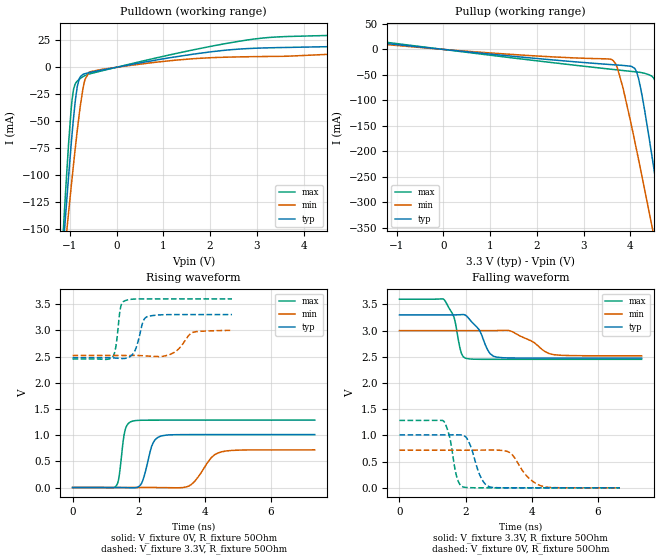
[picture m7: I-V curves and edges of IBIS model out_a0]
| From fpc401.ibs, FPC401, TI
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|   out_a0 Model
[Model]   out_a0
Model_type   Output
Polarity   Non-Inverting
Vmeas = 1.65
Vref = 0
Cref = 2pF
Rref = 5000
|   typ   min   max
|   (nom PVT)   (fast PVT)   (slow PVT)
C_comp   1.198e-12   1.173e-12   1.252e-12
| Where nom  PVT is Nominal Process, 3.3V, 27C
|   Fast PVT is Strong Process,  3.6V, -40C
|   Slow PVT is Weak Process,   3V, 125C
[Voltage Range]   3.3   3   3.6
|Junction Temperature
[Temperature Range]   27   125   -40
[Pullup Reference]   3.3   3   3.6
[Pulldown Reference]   0   0   0
[Power Clamp Reference]   3.3   3   3.6
[GND Clamp Reference]   0   0   0
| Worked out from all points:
|   slope of the pulldown table from 0 to 0.495 V, typ, clamps not added: 123 ohm
|   slope of the pullup table from 0 to 0.495 V, typ, clamps not added: 108 ohm
|   falling waveform, V_fixture 3.3V, R_fixture 50Ohm: 20-80 % time 426ps typ, 735ps min, 267ps max; typ from 3.3 V to 2.48 V
|   rising waveform, V_fixture 0V, R_fixture 50Ohm: 20-80 % time 249ps typ, 477ps min, 149ps max; typ from 0 V to 1.01 V
|   rising waveform, V_fixture 3.3V, R_fixture 50Ohm: 20-80 % time 209ps typ, 359ps min, 127ps max; typ from 2.48 V to 3.3 V
|   falling waveform, V_fixture 0V, R_fixture 50Ohm: 20-80 % time 317ps typ, 509ps min, 220ps max; typ from 1.01 V to 0 V
[Pulldown]
|   Voltage   I(typ)   I(min)   I(max)
-3.3V     -1.546A    -1.218A    -1.953A
-1.218V   -213.8mA   -220.6mA   -213.2mA
-1.115V   -152.3mA   -174.1mA   -133.9mA
-1.028V   -102.8mA   -136.1mA   -72.62mA
-924mV    -48.82mA   -91.83mA   -21.53mA
-838.2mV  -17.45mA   -58mA      -12.7mA
-696.3mV  -6.201mA   -15.06mA   -8.129mA
-582mV    -4.84mA    -4.296mA   -6.15mA
-330mV    -2.716mA   -2.011mA   -3.428mA
2.993V    17.77mA    9.963mA    26.56mA
4.584V    19.24mA    12.17mA    29.68mA
6.6V      33.13mA    35.22mA    33.6mA
[Pullup]
|   Voltage   I(typ)   I(min)   I(max)
-3.3V     32.44mA    31.14mA    37.81mA
3.585V    -29.8mA    -19.58mA   -38.89mA
3.726V    -30.71mA   -37.64mA   -40.28mA
4.029V    -33.53mA   -151.9mA   -43.21mA
4.175V    -56.83mA   -215.8mA   -44.69mA
4.454V    -204.9mA   -343.1mA   -52.13mA
4.518V    -242.7mA   -372.4mA   -59.95mA
4.591V    -287.3mA   -406.4mA   -92mA
4.663V    -331.4mA   -439.9mA   -139.5mA
4.749V    -384.4mA   -480mA     -203.1mA
4.937V    -501.6mA   -568mA     -351.5mA
6.6V      -1.559A    -1.368A    -1.735A
[Ramp]
R_load = 50
|   typ   min   max
dV/dt_r   0.605937/2.48756e-10   0.43132/4.77459e-10   0.77163/1.48535e-10
dV/dt_f   0.494035/4.25837e-10   0.288182/7.36969e-10   0.688486/2.66857e-10
[Falling Waveform]
V_fixture = 3.3V
V_fixture_min = 3V
V_fixture_max = 3.6V
R_fixture = 50Ohm
|   Time   V(typ)   V(min)   V(max)
0s        3.3V       3V         3.6V
1.352ns   3.3V       3V         3.591V
1.653ns   3.301V     3V         3.251V
1.877ns   3.305V     3V         2.561V
2.038ns   3.274V     3V         2.468V
2.433ns   2.993V     3V         2.453V
2.739ns   2.562V     3V         2.453V
2.951ns   2.494V     3.002V     2.453V
4.654ns   2.477V     2.542V     2.453V
7.325ns   2.477V     2.52V      2.453V
[Rising Waveform]
V_fixture = 0V
V_fixture_min = 0V
V_fixture_max = 0V
R_fixture = 50Ohm
|   Time   V(typ)   V(min)   V(max)
0s        1.218nV    15.44nV    982.1pV
1.311ns   439.2uV    480.9nV    25.22mV
1.586ns   -1.725mV   -17.86uV   1.089V
1.831ns   -5.716mV   27.74uV    1.27V
2.095ns   91.16mV    274.3uV    1.284V
2.39ns    782.6mV    301.2uV    1.286V
2.661ns   978.8mV    -772.7uV   1.286V
3.525ns   1.01V      30.92mV    1.286V
4.515ns   1.01V      682.6mV    1.286V
7.325ns   1.01V      718.9mV    1.286V
[Rising Waveform]
V_fixture = 3.3V
V_fixture_min = 3V
V_fixture_max = 3.6V
R_fixture = 50Ohm
|   Time   V(typ)   V(min)   V(max)
0s        2.477V     2.52V      2.453V
1.217ns   2.475V     2.52V      2.497V
1.311ns   2.47V      2.52V      2.695V
1.447ns   2.463V     2.52V      3.422V
1.586ns   2.464V     2.52V      3.565V
1.879ns   2.602V     2.52V      3.597V
2.257ns   3.26V      2.51V      3.6V
3.061ns   3.3V       2.573V     3.6V
3.634ns   3.3V       2.959V     3.6V
4.822ns   3.3V       2.999V     3.6V
[Falling Waveform]
V_fixture = 0V
V_fixture_min = 0V
V_fixture_max = 0V
R_fixture = 50Ohm
|   Time   V(typ)   V(min)   V(max)
0s        1.01V      718.9mV    1.286V
1.332ns   1.01V      718.9mV    1.277V
1.531ns   1.011V     718.9mV    934.8mV
1.753ns   1.012V     718.8mV    167.1mV
1.93ns    1.003V     718.7mV    16.23mV
2.492ns   162.8mV    720.7mV    419.7uV
2.739ns   15.94mV    722.1mV    142.9uV
3.327ns   442uV      676.2mV    20.68uV
4.298ns   5.386uV    34.54mV    7.334uV
6.669ns   11.05uV    -7.568uV   2.102uV
